(* Logix 5000 AddOnInstructionDefinition export; software revision 16.04 *)

ADD_ON_INSTRUCTION AMCI_ANG1E_Preset_Encoder_Position   (* revision 1.1, vendor AMCI *)
// Revision note:
// Version 1.1 added the slot_axis number and the input parameters can now be tags or discrete values.
VAR_INPUT
   slot_axis_number : DINT; {required}
   Target_Position : DINT; {required}
END_VAR
VAR_IN_OUT
   AMCI_ANG1E_output_data : INT[10]; {required}
END_VAR
VAR
   Upper_Result_X_1000 : DINT;
   command_data_block : INT[10];
        [0]   // Command Bits MSW
        [1]   // Command Bits LSW
        [2]   // Upper Target Position
        [3]   // Lower Target Position
        [4]   // Upper Programmed Speed
        [5]   // Lower Programmed Speed
   index : INT;
END_VAR

ROUTINE Logic   (* ladder *)
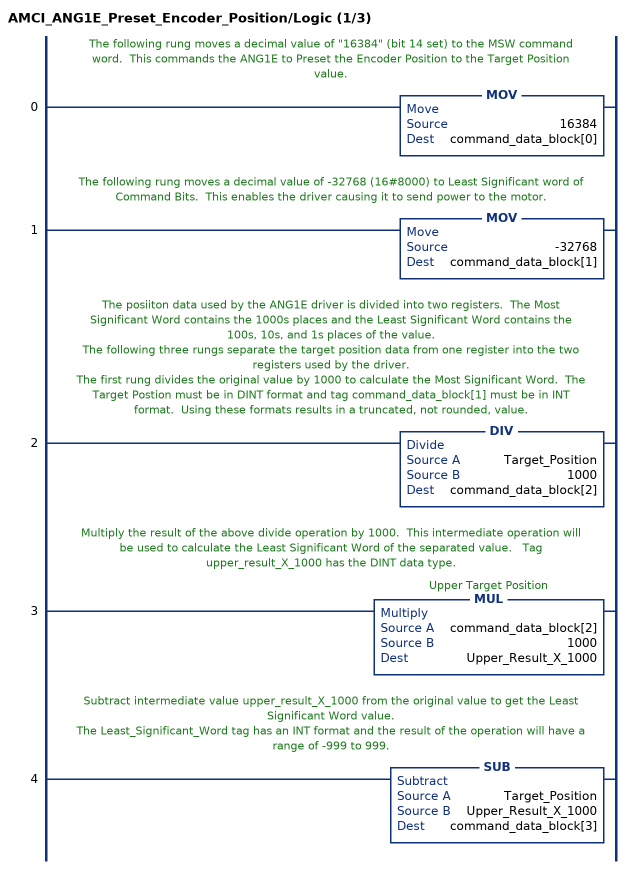
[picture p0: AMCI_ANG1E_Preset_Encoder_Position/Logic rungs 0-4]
   // The following rung moves a decimal value of "16384" (bit 14 set) to the MSW command word.  This commands the ANG1E to Preset the Encoder Position to the Target Position value.
   0: MOV(16384,command_data_block[0]);
   // The following rung moves a decimal value of -32768 (16#8000) to Least Significant word of Command Bits.  This enables the driver causing it to send power to the motor.
   1: MOV(-32768,command_data_block[1]);
   // The posiiton data used by the ANG1E driver is divided into two registers.  The Most Significant Word contains the 1000s places and the Least Significant Word contains the 100s, 10s, and 1s places of the value.
   // The following three rungs separate the target position data from one register into the two registers used by the driver.
   // The first rung divides the original value by 1000 to calculate the Most Significant Word.  The Target Postion must be in DINT format and tag command_data_block[1] must be in INT format.  Using these formats results in a truncated, not rounded, value.
   2: DIV(Target_Position,1000,command_data_block[2]);
   // Multiply the result of the above divide operation by 1000.  This intermediate operation will be used to calculate the Least Significant Word of the separated value.   Tag upper_result_X_1000 has the DINT data type.
   3: MUL(command_data_block[2],1000,Upper_Result_X_1000);
   // Subtract intermediate value upper_result_X_1000 from the original value to get the Least Significant Word value.
   // The Least_Significant_Word tag has an INT format and the result of the operation will have a range of -999 to 999.
   4: SUB(Target_Position,Upper_Result_X_1000,command_data_block[3]);
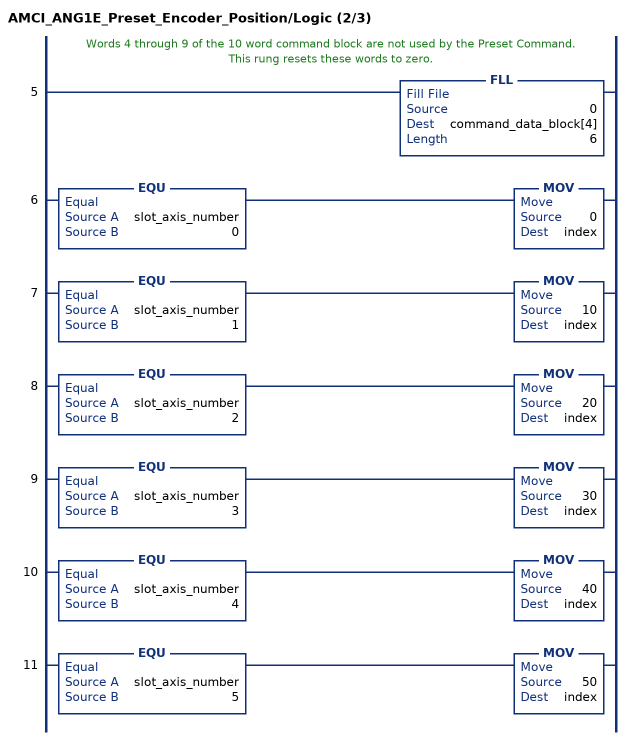
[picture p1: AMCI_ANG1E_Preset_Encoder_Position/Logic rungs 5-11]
   // Words 4 through 9 of the 10 word command block are not used by the Preset Command.  This rung resets these words to zero.
   5: FLL(0,command_data_block[4],6);
   6: EQU(slot_axis_number,0)MOV(0,index);
   7: EQU(slot_axis_number,1)MOV(10,index);
   8: EQU(slot_axis_number,2)MOV(20,index);
   9: EQU(slot_axis_number,3)MOV(30,index);
   10: EQU(slot_axis_number,4)MOV(40,index);
   11: EQU(slot_axis_number,5)MOV(50,index);
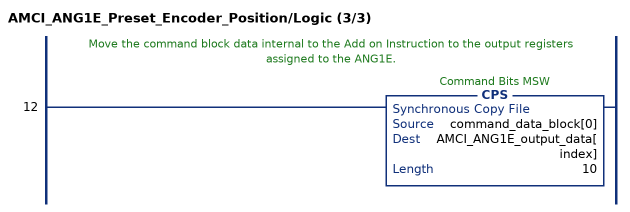
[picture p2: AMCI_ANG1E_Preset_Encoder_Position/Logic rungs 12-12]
   // Move the command block data internal to the Add on Instruction to the output registers assigned to the ANG1E.
   12: CPS(command_data_block[0],AMCI_ANG1E_output_data[index],10);
END_ROUTINE
END_ADD_ON_INSTRUCTION
